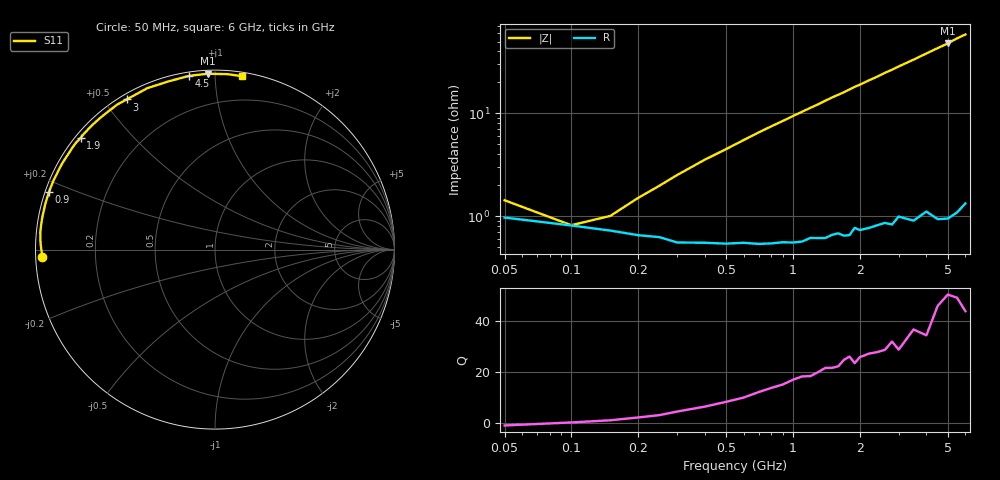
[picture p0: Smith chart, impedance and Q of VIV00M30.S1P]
! Infineon Technologies  Discrete & RF Semiconductors
! BB 804
! Si Tuning Diode in SOT23
! VR =
! S-Parameters:  July  1999
# GHz  S  MA  R  50
!  f  S11
! GHz  MAG  ANG
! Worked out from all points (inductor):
!   34 points, 50 MHz to 6 GHz, reference 50 ohm
!   read as one part to ground: L = 1.3 nH near 250 MHz
!   highest Q = 49.4 at 5 GHz (marker M1), where L = 1.53 nH
!   S11 on the Smith chart (normalised r, x): 50 MHz: 0.02, -0.02; 900 MHz: 0.01, +0.17; 1.9 GHz: 0.02, +0.36; 3 GHz: 0.02, +0.57; 4.5 GHz: 0.02, +0.86; 6 GHz: 0.03, +1.17
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0.05  0.962 -177.6
0.1  0.9681 179.8
0.2  0.9742 176.9
0.3  0.9781 174.4
0.4  0.9783 172.0
0.5  0.9788 169.8
0.7  0.9791 165.2
0.8  0.979 163.0
0.9  0.9786 160.9
1.1  0.9785 156.6
1.3  0.9772 152.5
1.5  0.976 148.2
1.6  0.9754 146.3
1.7  0.9769 144.4
1.8  0.9768 142.3
1.9  0.9732 140.2
2  0.9747 138.5
2.2  0.9742 134.6
2.4  0.9734 131.1
2.6  0.9728 127.3
2.8  0.9745 124.0
3  0.9706 120.5
3.5  0.9753 112.7
4  0.9724 105.2
4.5  0.9788 98.4
5  0.9805 92.4
5.5  0.98 86.0
6  0.9778 81.0
